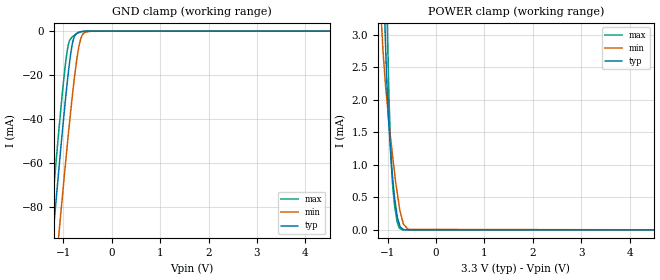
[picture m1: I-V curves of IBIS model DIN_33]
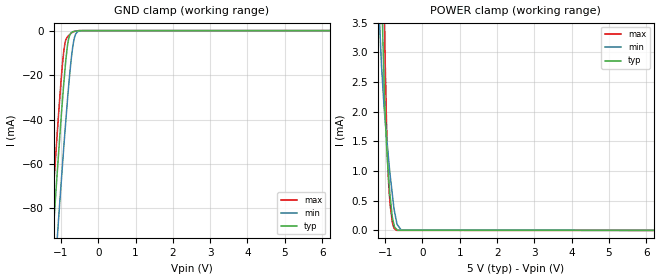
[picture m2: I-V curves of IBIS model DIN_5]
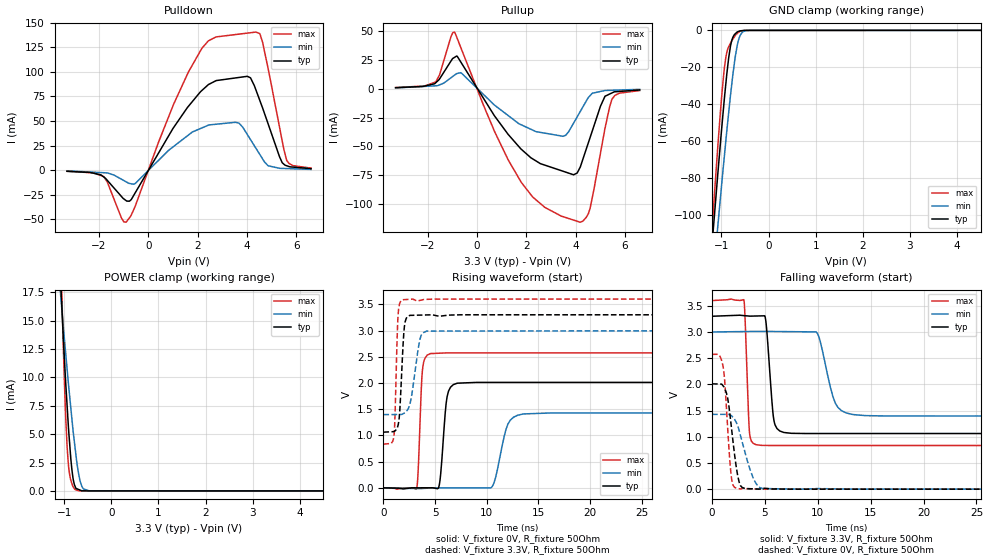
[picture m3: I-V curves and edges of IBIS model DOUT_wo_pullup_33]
|Texas Instruments Incorporated
|Ultra-Small, Low-Power, SPI-Compatible, 12-Bit
|Analog-to-Digital Converter and Temperature sesor
|with Internal Reference
| Marketing part#   Digital Voltage Range   Package-type   #pins
|ADS1018IDGSR   2V to 5.5V   MSOP   10
|ADS1018IDGST   2V to 5.5V   MSOP   10
|ADS1018IRUGR   2V to 5.5V   X2QFN   10
|ADS1018IRUGT   2V to 5.5V   X2QFN   10
[IBIS Ver]   4.0
[File name]   ads1018.ibs
[File Rev]   1.0
[Date]   11/16/2010
[Source]   Texas Instruments Incorporated.
   Analog-eLab, HPA
   12500 TI Blvd
   Dallas, TX -75243
   For Support e-mail: elab_ibis@list.ti.com
[Notes]   Revision History:
   1.0: 11/16/2010
   - Initial version of the model
   - Initial Model generated from simulations in TISPICED
   - Model names with a trailing _33 contains the model for
   3.3V (3.0V and 3.6V).
   _ Model names with trailing _5 contains
   the model for 5V (4.5V and 5.5V) operation.
   - Model not matched to measurements
[Disclaimer]
 This product is designed as an aid for customers of Texas Instruments.
 No warranties, either expressed or implied, with respect to this third
 party software (if any) or with respect to its fitness for any
 particular purpose is claimed by Texas Instruments or the author. The
 software (if any) is provided solely on an "as is" basis. The entire
 risk as to its quality and performance is with the customer
[Copyright] (C) Copyright 2012 Texas Instruments Incorporated.
   All rights reserved.
|   ADS1118
[Component]   ads1018rug
[Manufacturer] TI
[Package]   | 10 X2QFN - RUG package
| variable   typ   min   max
R_pkg  5.83238E-02   5.40400E-02   6.81900E-02
L_pkg  7.85773E-01nH 7.16980E-01nH 8.77680E-01nH
C_pkg  1.42156E-01pF 1.16570E-01pF 1.93520E-01pF
|-------------------------PIN------------------------------------------------
[Pin] signal_name  model_name  R_pin  L_pin C_pin
1   SCLK   DIN   0.06819   0.87719nH   0.12668pF
2   _CS   DIN   0.05404   0.77813nH   0.19312pF
3   GND   GND   0.05498   0.78912nH   0.19358pF
4   AIN0   TERM   0.05616   0.72411nH   0.11668pF
5   AIN1   TERM   0.05535   0.77700nH   0.13093pF
6   AIN2   TERM   0.05603   0.71698nH   0.11657pF
7   AIN3   TERM   0.05419   0.77463nH   0.19352pF
8   VDD   POWER   0.05623   0.79900nH   0.19475pF
9   DOUT_DRDY  DOUT   0.05950   0.76046nH   0.12056pF
10  DIN   DIN   0.06313   0.87768nH   0.13919pF
[Component]   ads1018dgs
[Manufacturer] TI
[Package]   | 10 MSOP - DGS package
| variable   typ   min   max
R_pkg  6.72725E-02   6.26300E-02   8.04000E-02
L_pkg  1.72557E+00nH 1.61576E+00nH 2.00802E+00nH
C_pkg  3.04549E-01pF 2.91740E-01pF 3.15100E-01pF
|-------------------------PIN------------------------------------------------
[Pin] signal_name  model_name  R_pin  L_pin C_pin
1   SCLK   DIN   0.08040   2.00802nH   0.30390pF
2   _CS   DIN   0.06263   1.62476nH   0.31385pF
3   GND   GND   0.06309   1.63746nH   0.31013pF
4   AIN0   TERM   0.06268   1.63079nH   0.31241pF
5   AIN1   TERM   0.06949   1.78291nH   0.29195pF
6   AIN2   TERM   0.06954   1.77442nH   0.29314pF
7   AIN3   TERM   0.06263   1.61576nH   0.31510pF
8   VDD   POWER   0.06311   1.62856nH   0.31029pF
9   DOUT_DRDY  DOUT   0.06295   1.62719nH   0.31430pF
10  DIN   DIN   0.06786   1.74072nH   0.29174pF
|   Model Selectors
[Model Selector]  DIN
DIN_33   3.3V digital input
DIN_5   5V digital input
|NOTES   Model DIN split into two Models DIN_33 and DIN_5
|   to accomodate vast voltage range of 2V - 5.5V
|   DIN_33 operates in voltage range of 3 - 3.3 - 3.6
|   DIN_5 operates in voltage range of 4.5 - 5 - 5.5
|   The max pin frequency for Model DIN is 10MHz.Also the
|   voltage range and frequency is referenced with datasheet.
[Model Selector]  DOUT
DOUT_w_pullup_33  3V digital output
DOUT_w_pullup_5  5V digital output
DOUT_wo_pullup_33  3V digital output
DOUT_wo_pullup_5  5V digital output
|NOTES   Model DOUT split into four Models DOUT_w_pullup_33,
|   DOUT_w_pullup_5, DOUT_wo_pullup_33, and DOUT_wo_pullup_5
|   to accomodate functionallity of this pin as well as the
|   vast voltage range of 2.7V - 5.5V. With these names,
|   w_pullup implies that bit 3 of the Config Registor is "0",
|   which disables the DOUT pin pulling it to DVDD with a
|   400 k ohm internal resistor. In this case DOUT in modeled as
|   an input buffer. If Bit 3 of the Config
|   Register is "1", DOUT funcitons as an output pin with
|   an internal tri-state conditions enabled with the
|   falling edge of chip select.
|   The DOUT symbol with a following _33 operates in voltage
|   range of 3 - 3.3 - 3.6. The DOUT symbol with a _5 at the end
|   of the buffer name operates in voltage range of 4.5 - 5 - 5.5.
|   The max pin frequency for Model DOUT is 10MHz.Also the
|   operation, voltage range, and frequency is referenced
|   with datasheet.
[Model Selector]  TERM
TERM_33  3V digital output
TERM_5  5V digital output
|   TERM Model
[Model] TERM_33
Model_type Terminator
C_comp   1e-20   1e-20   1e-20
| variable   typ   min   max
[Voltage Range]   3.3V   2.0V   5.5V
[POWER Clamp Reference]  3.3V   2.0V   5.5V
[GND Clamp Reference]   0.0V   0.0V   0.0V
|Operating Temperature   27   125   -40
[Temperature Range]   27   125   -40
|   TERM Model
[Model] TERM_5
Model_type Terminator
C_comp   1e-20   1e-20   1e-20
| variable   typ   min   max
[Voltage Range]   5V   4.5V   5.5V
[POWER Clamp Reference]  5V   4.5V   5.5V
[GND Clamp Reference]   0.0V   0.0V   0.0V
|Operating Temperature   27   125   -40
[Temperature Range]   27   125   -40
| Models and submodels in the file (8): DIN_33 (Input), DIN_5 (Input), DOUT_wo_pullup_33 (3-state), DOUT_w_pullup_33 (3-state), DOUT_wo_pullup_5 (3-state), DOUT_w_pullup_5 (3-state), TERM_33 (Terminator), TERM_5 (Terminator)
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|NOTES   Model TERM split into two Models TERM_33 and TERM_5
|   to accomodate vast voltage range of 2.7V - 5.5V
|   TERM_33 operates in voltage range of 3 - 3.3 - 3.6
|   TERM_5 operates in voltage range of 4.5 - 5 - 5.5
|   DIN Model
[Model] DIN_33
|  Signals SCLK(1), _CS(2), DIN(10)
Model_type Input
Vinl = 0.99
Vinh = 2.31
|   typ   min   max
|   (nom PVT)   (Fast PVT)   (slow PVT)
C_comp   1.2687330e-12  1.0858990e-12  1.4598910e-12
| Where   nom PVT is  Nominal Process, 3.3V, 27C
|   Fast PVT is Strong or Fast Process, 3.6V, -40C
|   Slow PVT is Weak or slow Process, 3.0V, 125C
| variable   typ   min   max
[Voltage Range]   3.3   3   3.6
|Operating Temperature   27   125   -40
[Temperature Range]   27   125   -40
[Power Clamp Reference]   3.3   3   3.6
[GND Clamp Reference]   0   0   0
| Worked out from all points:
|   GND clamp passes 1 mA (typ) near -0.72 V on its own axis
|   POWER clamp passes 1 mA (typ) near -0.92 V on its own axis
[GND Clamp]
|   Voltage   I(typ)   I(min)   I(max)
-3.3V     -642.4mA   -658.9mA   -636.4mA
-1.283V   -109.1mA   -137.9mA   -92.24mA
-1.226V   -94.93mA   -123.9mA   -77.64mA
-1.178V   -82.78mA   -112.1mA   -65.38mA
-1.089V   -60.97mA   -90.57mA   -43.35mA
-931.6mV  -25.16mA   -53.95mA   -10.15mA
-882.9mV  -15.68mA   -43.22mA   -4.889mA
-817.5mV  -5.824mA   -29.48mA   -2.626mA
-699.2mV  -630.2uA   -9.124mA   -854.9uA
-600mV    -134.4uA   -1.376mA   -206.6uA
-419.4mV  -17.66uA   -16.11uA   -22.09uA
6.6V      0A         0A         0A
[POWER Clamp]
|   Voltage   I(typ)   I(min)   I(max)
-3.3V     95.3mA     72.1mA     119.4mA
-1.12V    4.851mA    3.072mA    7.597mA
-1.057V   3.145mA    2.349mA    4.936mA
-1.019V   2.303mA    2.014mA    3.497mA
-983.7mV  1.713mA    1.728mA    2.35mA
-941mV    1.21mA     1.412mA    1.308mA
-892.1mV  755.6uA    1.097mA    637.8uA
-854.5mV  477.2uA    854.4uA    360.1uA
-800mV    193.8uA    559uA      116.7uA
-697.2mV  20.7uA     154.3uA    2.443uA
-576.2mV  3.811uA    8.235uA    2.403uA
6.6V      0A         0A         0A
|   DIN Model
[Model] DIN_5
|  Signals SCLK(1), _CS(2), DIN(10)
Model_type Input
Vinl = 1.5
Vinh = 3.5
|   typ   min   max
|   (nom PVT)   (Fast PVT)   (slow PVT)
C_comp   1.1865890e-12  1.0211560e-12  1.3385550e-12
| Where   nom PVT is  Nominal Process, 5V, 27C
|   Fast PVT is Strong or Fast Process, 5.5V, -40C
|   Slow PVT is Weak or Slow Process, 4.5V, 125C
[Voltage Range]   5   4.5   5.5
|Operating Temperature   27   125   -40
[Temperature Range]   27   125   -40
[Power Clamp Reference]   5   4.5   5.5
[GND Clamp Reference]   0   0   0
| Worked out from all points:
|   GND clamp passes 1 mA (typ) near -0.72 V on its own axis
|   POWER clamp passes 1 mA (typ) near -0.92 V on its own axis
[GND Clamp]
|   Voltage   I(typ)   I(min)   I(max)
-5V       -1.099A    -1.107A    -1.101A
-1.274V   -107mA     -135.8mA   -89.9mA
-1.225V   -94.69mA   -123.8mA   -77.53mA
-1.177V   -82.6mA    -111.8mA   -65.08mA
-1.083V   -59.66mA   -89.2mA    -41.86mA
-922.9mV  -23.44mA   -51.94mA   -8.91mA
-880.1mV  -15.08mA   -42.64mA   -4.709mA
-810.1mV  -5.06mA    -27.95mA   -2.509mA
-690.7mV  -545.9uA   -8.066mA   -779.2uA
-603mV    -281.9uA   -1.473mA   -213.7uA
-410.1mV  -10.91uA   -12.45uA   -17.5uA
10V       0A         0A         0A
[POWER Clamp]
|   Voltage   I(typ)   I(min)   I(max)
-5V       168.8mA    130.5mA    208.9mA
-1.161V   6.153mA    3.658mA    9.424mA
-1.135V   5.315mA    3.288mA    8.228mA
-1.064V   3.275mA    2.43mA     5.204mA
-1.016V   2.239mA    1.972mA    3.389mA
-955.9mV  1.358mA    1.54mA     1.618mA
-902.6mV  848.8uA    1.163mA    744.2uA
-860.1mV  531.2uA    895.7uA    394uA
-812.3mV  247.9uA    632uA      159.1uA
-693.3mV  20.2uA     139.4uA    2.078uA
-571.2mV  3.883uA    7.176uA    2.054uA
10V       0A         0A         0A
|   DOUT Model 3.3 V model  Config Register bit3=1
[Model] DOUT_wo_pullup_33
|  Signals  DOUT/_DRDY(9)
|   bit 3 of the Config Registor is one
Model_type 3-state
Polarity   Non-Inverting
Enable   Active-Low
Vmeas = 1.65
Vref = 1.65
Cref = 15pF
Rref = 50
|   typ   min   max
|   (nom PVT)   (Fast PVT)   (slow PVT)
C_comp   2.0567970e-12  1.6524170e-12  2.4825130e-12
|   typ   min   max
|   (Fast PVT)   (nom PVT)   (slow PVT)
|C_comp (ON state)   2.9653630e-12  2.6925520e-12  3.3967920e-12
|C_comp (OFF state)   3.0077420e-12  2.9299510e-12  3.3223790e-12
| Where   nom PVT is  Nominal Process, 3.3V, 27C
|   Fast PVT is Strong or Fast Process, 3.6V, -40C
|   Slow PVT is Weak or slow Process, 3.0V, 125C
[Voltage Range]   3.3   3   3.6
|Operating Temperature   27   125   -40
[Temperature Range]   27   125   -40
[Pullup Reference]   3.3   3   3.6
[Pulldown Reference]   0   0   0
[Power Clamp Reference]   3.3   3   3.6
[GND Clamp Reference]   0   0   0
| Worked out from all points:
|   slope of the pulldown table from 0 to 0.495 V, typ, clamps not added: 23.4 ohm
|   slope of the pullup table from 0 to 0.495 V, typ, clamps not added: 29.3 ohm
|   GND clamp passes 1 mA (typ) near -0.67 V on its own axis
|   POWER clamp passes 1 mA (typ) near -0.81 V on its own axis
|   falling waveform, V_fixture 3.3V, R_fixture 50Ohm: 20-80 % time 490ps typ, 1.12ns min, 297ps max; typ from 3.3 V to 1.06 V
|   rising waveform, V_fixture 0V, R_fixture 50Ohm: 20-80 % time 469ps typ, 957ps min, 305ps max; typ from 0 V to 2.01 V
|   rising waveform, V_fixture 3.3V, R_fixture 50Ohm: 20-80 % time 347ps typ, 699ps min, 239ps max; typ from 1.06 V to 3.3 V
|   falling waveform, V_fixture 0V, R_fixture 50Ohm: 20-80 % time 726ps typ, 1.23ns min, 495ps max; typ from 2.01 V to 0 V
[Pulldown]
|   Voltage   I(typ)   I(min)   I(max)
-3.3V     -1.144mA   -709uA     -1.168mA
-1.814V   -6.852mA   -2.607mA   -6.413mA
-903.7mV  -30.91mA   -11.83mA   -52.9mA
-531.3mV  -23.01mA   -13.54mA   -36.63mA
1.037V    43.74mA    24.31mA    67.65mA
2.166V    80.87mA    42.85mA    123.6mA
3.679V    94.24mA    47.75mA    138.3mA
4.145V    93.85mA    31.03mA    139.7mA
4.357V    82mA       22.53mA    140.4mA
4.633V    63.31mA    11.5mA     130.2mA
5.604V    4.535mA    1.623mA    10.52mA
6.6V      1.521mA    772.7uA    2.055mA
[GND Clamp]
|   Voltage   I(typ)   I(min)   I(max)
-3.3V     -822.2mA   -770.1mA   -947.3mA
-1.206V   -117.8mA   -142mA     -109.7mA
-1.171V   -106.9mA   -132.3mA   -96.92mA
-1.077V   -77.5mA    -105.7mA   -62.66mA
-981.2mV  -49.08mA   -79.32mA   -31.51mA
-911.9mV  -30.13mA   -61.04mA   -15.45mA
-848.6mV  -15.34mA   -45.03mA   -9.041mA
-793.4mV  -6.742mA   -31.87mA   -6.114mA
-662.9mV  -866.7uA   -7.886mA   -1.636mA
-575.5mV  -203.6uA   -1.602mA   -385.4uA
-402.3mV  -26.17uA   -18.95uA   -47.08uA
6.6V      0A         0A         0A
[Pullup]
|   Voltage   I(typ)   I(min)   I(max)
-3.3V     826uA      588.9uA    924.3uA
-1.674V   5.029mA    2.454mA    5.742mA
-920.3mV  26.88mA    11.52mA    48.86mA
-625.3mV  21.96mA    13.32mA    33.86mA
726.2mV   -23.98mA   -14.49mA   -37.65mA
1.788V    -52.21mA   -31.18mA   -80.65mA
3.497V    -71.44mA   -41.17mA   -110.7mA
4.184V    -68.02mA   -19.99mA   -115.4mA
4.583V    -42.59mA   -6.194mA   -103.8mA
5.19V     -6.713mA   -1.635mA   -34.61mA
5.469V    -3.782mA   -1.422mA   -9.509mA
6.6V      -1.155mA   -649.9uA   -1.664mA
[POWER Clamp]
|   Voltage   I(typ)   I(min)   I(max)
-3.3V     274.7mA    182.6mA    430.3mA
-1.077V   18.65mA    17.34mA    21.4mA
-1.049V   16.16mA    15.93mA    17.05mA
-990.1mV  11.23mA    13.11mA    9.006mA
-937.5mV  7.451mA    10.69mA    3.846mA
-903.7mV  5.211mA    9.162mA    2.03mA
-857.8mV  2.752mA    7.242mA    928.7uA
-768.3mV  395uA      3.774mA    120.8uA
-703mV    142.3uA    1.724mA    31.16uA
-625.3mV  8.422uA    396.8uA    10.33uA
-465.5mV  5.206uA    5.5uA      10.1uA
6.6V      0A         0A         0A
[Ramp]
R_load = 50
|   typ   min   max
dV/dt_r   1.2062/4.66181e-010   0.8568/9.4597e-010   1.54377/3.0446e-010
dV/dt_f   1.34314/4.86565e-010  0.962561/1.11297e-009   1.66033/2.94412e-010
[Falling Waveform]
V_fixture = 3.3V
V_fixture_min = 3V
V_fixture_max = 3.6V
R_fixture = 50Ohm
C_fixture = 0F
|   Time   V(typ)   V(min)   V(max)
0s        3.3V       3V         3.6V
3.008ns   3.313V     3.008V     3.617V
3.537ns   3.303V     3.009V     1.093V
4.158ns   3.305V     3.011V     848.9mV
5.019ns   3.289V     3.011V     835mV
5.836ns   1.331V     3.009V     833mV
6.789ns   1.082V     3.007V     833mV
9.924ns   1.062V     2.984V     832.9mV
13.31ns   1.062V     1.424V     832.9mV
50ns      1.061V     1.396V     832.8mV
[Rising Waveform]
V_fixture = 0V
V_fixture_min = 0V
V_fixture_max = 0V
R_fixture = 50Ohm
C_fixture = 0F
|   Time   V(typ)   V(min)   V(max)
0s        589.3pV    1.019nV    505.3pV
3.219ns   -528.8uV   -13.94mV   -14.39mV
3.785ns   -231.4uV   -13.14mV   2.248V
4.54ns    165.4uV    -4.043mV   2.559V
5.358ns   10.84mV    -773.3uV   2.567V
6.164ns   1.733V     -979.3uV   2.573V
7.152ns   1.995V     -1.232mV   2.573V
10.51ns   2.01V      15.92mV    2.573V
13.54ns   2.01V      1.409V     2.573V
50ns      2.01V      1.428V     2.573V
[Rising Waveform]
V_fixture = 3.3V
V_fixture_min = 3V
V_fixture_max = 3.6V
R_fixture = 50Ohm
C_fixture = 0F
|   Time   V(typ)   V(min)   V(max)
0s        1.061V     1.396V     832.8mV
1.016ns   1.071V     1.398V     983.2mV
1.421ns   1.194V     1.399V     3.291V
1.594ns   1.5V       1.399V     3.526V
1.884ns   2.651V     1.41V      3.587V
2.21ns    3.232V     1.455V     3.591V
2.719ns   3.29V      1.738V     3.598V
3.559ns   3.294V     2.846V     3.575V
4.185ns   3.297V     2.989V     3.594V
50ns      3.3V       3V         3.6V
[Falling Waveform]
|Gnd
V_fixture = 0V
V_fixture_min = 0V
V_fixture_max = 0V
R_fixture = 50Ohm
C_fixture = 0F
|   Time   V(typ)   V(min)   V(max)
0s        2.01V      1.428V     2.573V
1.037ns   1.974V     1.427V     2.348V
1.209ns   1.912V     1.427V     2.034V
1.479ns   1.736V     1.427V     1.16V
1.808ns   1.221V     1.405V     261.4mV
2.339ns   362mV      1.252V     14.06mV
2.694ns   66.35mV    1.018V     5.448mV
3.846ns   6.358mV    235.8mV    4.713mV
4.837ns   12.26mV    11.59mV    342uV
50ns      589.3pV    1.019nV    505.3pV
